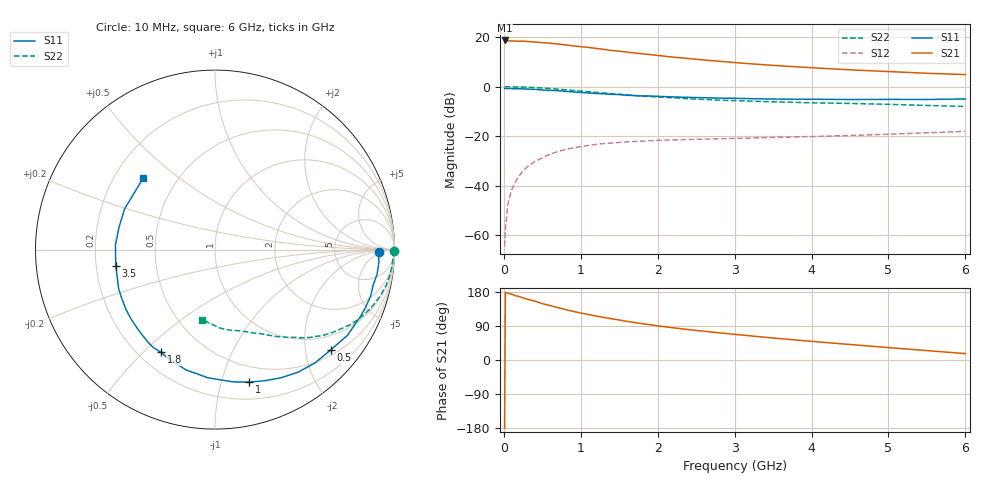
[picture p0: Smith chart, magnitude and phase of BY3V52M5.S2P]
! SIEMENS Small Signal Semiconductors
! BFY420
! Si NPN RF SIEGET Grounded Emitter Transistor in MICRO-X
! VCE = 3.5 V  IC = 2.5 mA
! Common Emitter S-Parameters:  October  1996
# GHz  S  MA  R  50
!  f  S11  S21  S12  S22
! GHz  MAG  ANG  MAG  ANG  MAG  ANG  MAG  ANG
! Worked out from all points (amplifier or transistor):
!   36 points, 10 MHz to 6 GHz, reference 50 ohm
!   highest |S21| = 18.6 dB at 10 MHz (marker M1)
!   |S21| within 3 dB of that: start of sweep to 1.149 GHz
!   unconditionally stable (mu >= 1): 3.811 GHz to end of sweep
!   at 250 MHz: K = 0.09, MSG = 26.2 dB, |S12| = -34.0 dB
!   at 1.4 GHz: K = 0.33, MSG = 18.7 dB, |S12| = -22.8 dB
!   at 6 GHz: K = 1.20, MAG = 8.8 dB, |S12| = -18.1 dB
!   S11 on the Smith chart (normalised r, x): 10 MHz: 21, -4; 500 MHz: 0.62, -2.55; 1 GHz: 0.35, -1.23; 1.8 GHz: 0.29, -0.57; 3.5 GHz: 0.28, -0.07; 6 GHz: 0.32, +0.38
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0.01  0.9131 -1.0  8.546 -179.8  0.0006 79.0  0.9961 -0.4
0.02  0.9116 -1.8  8.537 178.2  0.0013 75.9  0.9924 -0.8
0.05  0.916 -4.3  8.349 176.2  0.0041 82.7  0.9938 -2.0
0.1  0.9135 -8.6  8.362 173.9  0.0081 82.5  0.9918 -4.0
0.15  0.9033 -12.5  8.293 169.7  0.0119 79.8  0.9885 -6.0
0.2  0.9047 -16.7  8.274 167.5  0.0158 80.7  0.9857 -7.9
0.25  0.8983 -21.1  8.28 164.0  0.02 75.9  0.9787 -10.0
0.4  0.8788 -33.0  7.957 155.5  0.0304 71.3  0.9561 -15.7
0.5  0.8534 -40.9  7.715 148.7  0.0367 67.3  0.9352 -19.2
0.7  0.8255 -55.7  7.261 138.4  0.0486 59.5  0.8886 -25.9
0.8  0.8032 -62.8  6.955 133.2  0.0537 55.3  0.863 -28.9
1  0.7624 -75.6  6.407 124.1  0.0613 49.6  0.812 -34.0
1.1  0.7439 -82.2  6.19 120.0  0.0649 47.2  0.7882 -36.5
1.4  0.6985 -98.5  5.376 108.8  0.0726 40.4  0.7217 -42.7
1.6  0.6694 -109.1  4.96 101.9  0.0766 37.0  0.68 -46.3
1.8  0.6465 -117.7  4.589 95.8  0.0793 33.9  0.647 -49.1
2.2  0.6192 -133.3  3.933 85.1  0.084 29.5  0.5947 -54.6
2.8  0.5861 -152.6  3.252 71.7  0.0886 25.5  0.5327 -61.5
3.5  0.5601 -170.7  2.68 58.0  0.094 23.3  0.493 -68.5
4.5  0.549 166.5  2.18 40.9  0.103 21.3  0.4572 -79.3
5.5  0.5495 145.3  1.856 24.8  0.1167 19.7  0.4157 -92.7
6  0.564 135.2  1.749 16.9  0.1249 18.4  0.3977 -100.5
